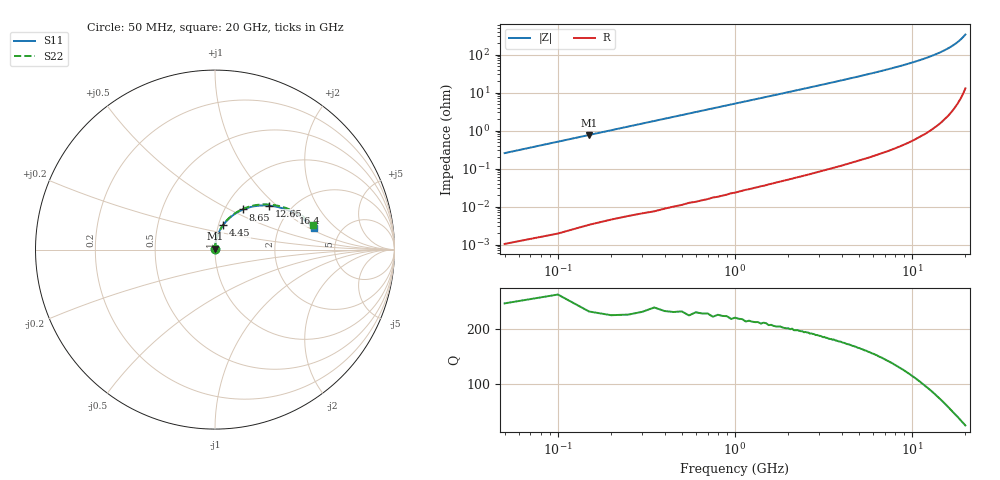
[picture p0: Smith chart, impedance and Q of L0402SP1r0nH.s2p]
!	AVX Thin Film Operation
!	Date:		5 January 2004
!	Description: 	Accu-L®  L0402 Series Thin Film RF Inductors
!	Part Number:	L04021R0AHLTR
!	50 MHz-20GHz Serial Measurements
#	mhz	S	db	R	50
!	S11	S11	S21	S21	S12	S12	S22	S22
!	dB	Phase	dB	Phase	dB	Phase	dB	Phase
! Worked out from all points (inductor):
!   400 points, 50 MHz to 20 GHz, reference 50 ohm
!   read as 1/Y11, port 2 shorted: L = 812 pH near 150 MHz
!   highest Q = 238 at 150 MHz (marker M1), where L = 812 pH
!   S11 on the Smith chart (normalised r, x): 50 MHz: 1.00, +0.00; 4.45 GHz: 1.05, +0.29; 8.65 GHz: 1.22, +0.59; 12.65 GHz: 1.54, +0.89; 16.4 GHz: 2.14, +1.14; 20 GHz: 3.16, +1.09
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50  -55.77 89.4  -0.00 -0.2  -0.00 -0.2  -55.77 89.4
100  -49.75 89.2  -0.00 -0.4  -0.00 -0.4  -49.75 89.2
150  -46.23 89.0  -0.00 -0.6  -0.00 -0.6  -46.23 89.0
200  -43.73 88.8  -0.00 -0.8  -0.00 -0.8  -43.73 88.8
250  -41.79 88.6  -0.00 -1.0  -0.00 -1.0  -41.79 88.6
350  -38.87 88.2  -0.00 -1.4  -0.00 -1.4  -38.87 88.2
450  -36.68 87.8  -0.00 -1.8  -0.00 -1.8  -36.68 87.8
700  -32.85 86.8  -0.00 -2.8  -0.00 -2.8  -32.85 86.9
1050  -29.32 85.4  -0.01 -4.2  -0.01 -4.2  -29.32 85.5
1450  -26.52 83.7  -0.01 -5.8  -0.01 -5.8  -26.52 83.9
2000  -23.73 81.5  -0.02 -8.0  -0.02 -8.0  -23.73 81.7
2650  -21.30 78.9  -0.04 -10.5  -0.04 -10.5  -21.30 79.1
3400  -19.15 75.8  -0.06 -13.5  -0.06 -13.5  -19.15 76.2
4450  -16.84 71.6  -0.10 -17.7  -0.10 -17.7  -16.84 72.0
6700  -13.37 62.6  -0.22 -26.5  -0.22 -26.5  -13.37 63.3
8650  -11.25 54.8  -0.36 -34.1  -0.36 -34.1  -11.25 55.7
10050  -10.04 49.3  -0.48 -39.5  -0.48 -39.5  -10.04 50.3
12650  -8.24 39.3  -0.75 -49.4  -0.75 -49.4  -8.24 40.5
13350  -7.83 36.6  -0.83 -52.0  -0.83 -52.0  -7.83 37.9
16400  -6.33 25.1  -1.22 -63.3  -1.22 -63.3  -6.33 26.7
16700  -6.20 24.0  -1.26 -64.4  -1.26 -64.4  -6.20 25.6
20000  -4.99 12.1  -1.75 -76.1  -1.75 -76.1  -4.99 14.0
